FUNCTION_BLOCK Example09_groupstatus //2x1 flyways 2 xbots - delete group, get group status, get macro status
VAR_INPUT
	Execute : BOOL;
END_VAR
VAR_OUTPUT
	Done : BOOL;
END_VAR
VAR_IN_OUT
	PM_Controller : PMControllerType;	// the planar motor controller to use
END_VAR
VAR
	xbotID_array32 : ARRAY[0..31] OF USINT;
	PMC_CreateXbotGroup1 : PMC_CreateXbotGroup;
	group_state1 : USINT;
	nxbots1 : USINT;
	return_xbotID_array1 : ARRAY[0..31] OF USINT;
	PMC_GetGroupStatus1 : PMC_GetGroupStatus;
	PMC_BondXbotGroup1 : PMC_BondXbotGroup;
	group_state2 : USINT;
	nxbots2 : USINT;
	return_xbotID_array2 : ARRAY[0..31] OF USINT;
	PMC_GetGroupStatus2 : PMC_GetGroupStatus;
	PMC_DeleteXbotGroup1 : PMC_DeleteXbotGroup;
	group_state3 : USINT;
	nxbots3 : USINT;
	return_xbotID_array3 : ARRAY[0..31] OF USINT;
	PMC_GetGroupStatus3 : PMC_GetGroupStatus;
	PMC_ClearMacro1 : PMC_ClearMacro;
	macro_state1 : USINT;
	nCmds1 : UINT;
	PMC_GetMacroStatus1 : PMC_GetMacroStatus;
	PMC_XYMotion1 : PMC_XYMotion;
	PMC_XYMotion2 : PMC_XYMotion;
	PMC_SaveMacro1 : PMC_SaveMacro;
	macro_state2 : USINT;
	nCmds2 : UINT;
	PMC_GetMacroStatus2 : PMC_GetMacroStatus;
END_VAR

//2x1 flyways 2 xbots - delete group, get group status, get macro status

//create group 1 from xbot 1 and 2
xbotID_array32[0] := 1;xbotID_array32[1] := 2;
PMC_CreateXbotGroup1(Execute := Execute,GroupID := 1,nXbots := 2,XbotID := xbotID_array32,PM_Controller := PM_Controller);

//get status of group 1
PMC_GetGroupStatus1(Execute := PMC_CreateXbotGroup1.Done,GroupID := 1,State => group_state1,nXbots => nxbots1,XbotID => return_xbotID_array1,PM_Controller := PM_Controller);

//bond group 1
PMC_BondXbotGroup1(Execute := PMC_GetGroupStatus1.Done,GroupID := 1,IsBond := TRUE,Mode := 0,PM_Controller := PM_Controller);

//get status of group 1
PMC_GetGroupStatus2(Execute := PMC_BondXbotGroup1.Done,GroupID := 1,State => group_state2,nXbots => nxbots2,XbotID => return_xbotID_array2,PM_Controller := PM_Controller);

//delete group 1
PMC_DeleteXbotGroup1(Execute := PMC_GetGroupStatus2.Done,GroupID := 1,PM_Controller := PM_Controller);

//get status of group 1
PMC_GetGroupStatus3(Execute := PMC_DeleteXbotGroup1.Done,GroupID := 1,State => group_state3,nXbots => nxbots3,XbotID => return_xbotID_array3,PM_Controller := PM_Controller);

//clear macro 128
PMC_ClearMacro1(Execute := PMC_GetGroupStatus3.Done,MacroID := 128,PM_Controller := PM_Controller);

//get status of macro 128
PMC_GetMacroStatus1(Execute := PMC_ClearMacro1.Done,MacroID := 128,State => macro_state1,nCmds => nCmds1,PM_Controller := PM_Controller);

//add command to macro 128
PMC_XYMotion1(Execute := PMC_GetMacroStatus1.Done,cmdLB := 9,XbotID := 128,Mode := 0,Type_ := 0,PosX := 0.9,PosY := 0.06,EndVel := 0,MaxVel := 1,MaxAcc := 10,PM_Controller := PM_Controller);

//add command to macro 128
PMC_XYMotion2(Execute := PMC_XYMotion1.Done,cmdLB := 10,XbotID := 128,Mode := 0,Type_ := 0,PosX := 0.06,PosY := 0.06,EndVel := 0,MaxVel := 1,MaxAcc := 10,PM_Controller := PM_Controller);

//save macro 128
PMC_SaveMacro1(Execute := PMC_XYMotion2.Done,MacroID := 128,PM_Controller := PM_Controller);

//get status of macro 128
PMC_GetMacroStatus2(Execute := PMC_SaveMacro1.Done,MacroID := 128,State => macro_state2,nCmds => nCmds2,PM_Controller := PM_Controller);

Done := PMC_GetMacroStatus2.Done;

END_FUNCTION_BLOCK
